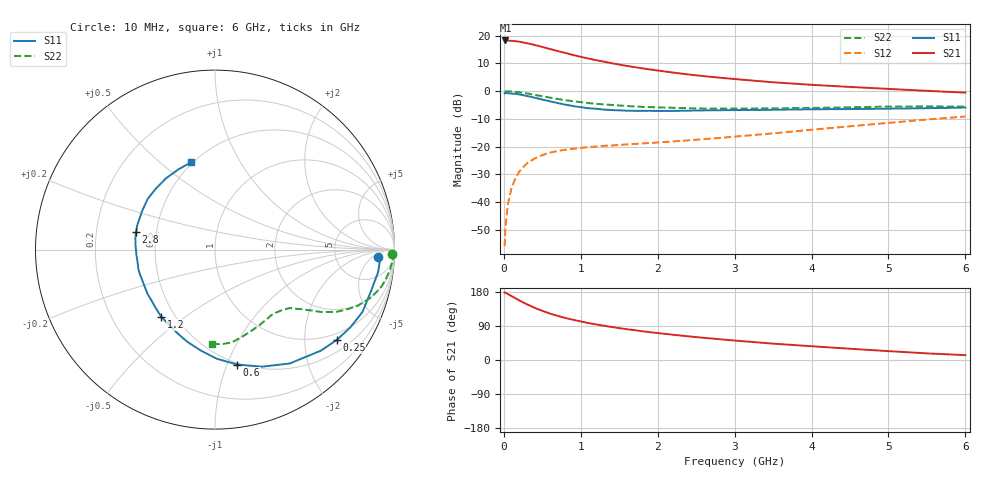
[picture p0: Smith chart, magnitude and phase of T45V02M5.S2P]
! Infineon Technologies  Discrete & RF Semiconductors
! BFR182T
! Si NPN RF Bipolar Junction Transistor in SC75
! VCE = 5 V  IC = 2.5 mA
! Common Emitter S-Parameters:  October  1999
# GHz  S  MA  R  50
!  f  S11  S21  S12  S22
! GHz  MAG  ANG  MAG  ANG  MAG  ANG  MAG  ANG
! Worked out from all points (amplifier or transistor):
!   36 points, 10 MHz to 6 GHz, reference 50 ohm
!   highest |S21| = 18.2 dB at 20 MHz (marker M1)
!   |S21| within 3 dB of that: start of sweep to 588.3 MHz
!   unconditionally stable (mu >= 1): 1.893 GHz to 4.278 GHz
!   at 250 MHz: K = 0.16, MSG = 22.5 dB, |S12| = -27.5 dB
!   at 1.4 GHz: K = 0.83, MSG = 14.8 dB, |S12| = -19.6 dB
!   at 6 GHz: K = 0.83, MSG = 4.3 dB, |S12| = -9.2 dB
!   lowest NFmin = 1.10 dB at 450 MHz
!   S11 on the Smith chart (normalised r, x): 10 MHz: 17, -8; 250 MHz: 0.80, -2.82; 600 MHz: 0.49, -1.09; 1.2 GHz: 0.42, -0.41; 2.8 GHz: 0.38, +0.10; 6 GHz: 0.49, +0.64
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0.01  0.9069 -2.6  8.113 178.1  0.0016 78.9  0.9873 -1.4
0.02  0.924 -1.9  8.16 177.9  0.0033 103.4  0.9858 -1.2
0.05  0.9175 -7.8  8.135 174.1  0.0088 87.4  0.9918 -3.2
0.1  0.8995 -14.9  8.018 168.8  0.018 82.7  0.9824 -6.4
0.15  0.8922 -22.9  7.926 162.9  0.0266 77.7  0.968 -9.4
0.25  0.8446 -36.6  7.525 152.2  0.0423 70.4  0.9288 -14.9
0.3  0.8153 -43.7  7.278 147.1  0.0496 67.6  0.9063 -17.3
0.4  0.759 -56.7  6.774 137.7  0.0608 61.5  0.8544 -21.5
0.5  0.703 -68.1  6.232 129.8  0.0701 56.9  0.805 -24.5
0.6  0.652 -79.1  5.719 122.5  0.0776 52.6  0.7606 -27.1
0.8  0.5684 -97.9  4.852 110.9  0.0876 48.1  0.6844 -30.5
0.9  0.5362 -106.8  4.464 106.1  0.0907 46.3  0.6538 -31.6
1.1  0.4903 -122.0  3.86 97.4  0.0978 44.6  0.6082 -33.5
1.2  0.4793 -128.6  3.6 94.0  0.0999 44.0  0.5883 -34.4
1.4  0.4537 -141.2  3.173 87.2  0.1042 43.9  0.5619 -36.0
1.6  0.4424 -152.7  2.834 81.2  0.1092 44.4  0.5371 -37.4
2.2  0.4389 -176.3  2.153 66.6  0.1234 48.6  0.4991 -43.1
2.8  0.451 167.2  1.743 54.9  0.1425 53.1  0.4814 -50.1
3.5  0.4596 151.9  1.439 43.2  0.1728 57.0  0.4875 -58.8
4.5  0.4732 134.4  1.186 29.7  0.2317 58.8  0.5089 -72.7
5.5  0.4909 114.9  1.009 17.5  0.3065 56.3  0.5284 -85.9
6  0.5042 105.5  0.936 12.8  0.348 53.4  0.5251 -91.8
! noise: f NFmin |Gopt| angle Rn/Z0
0.45  1.1  0.39  29  0.35
0.9  1.2  0.37  59  0.28
1.8  1.8  0.28  128  0.2
